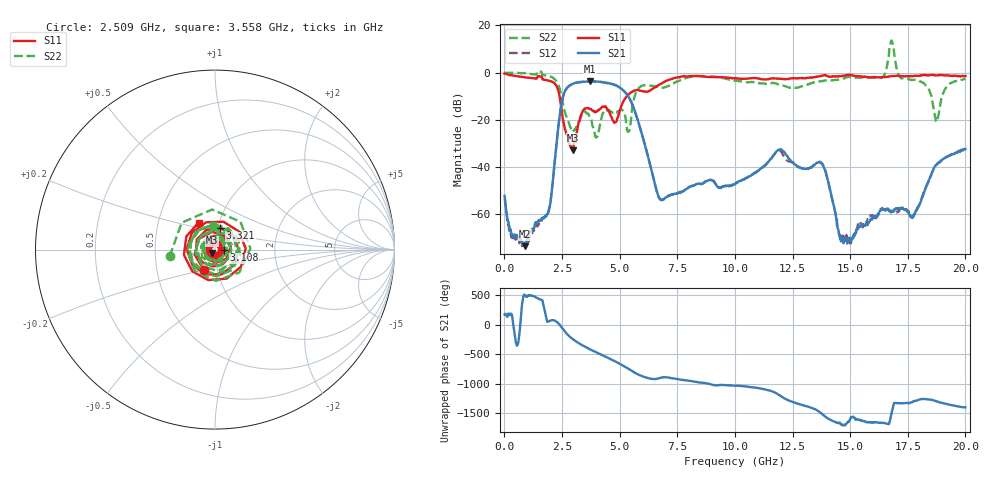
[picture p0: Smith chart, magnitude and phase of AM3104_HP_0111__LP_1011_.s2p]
!Created with skrf (http://scikit-rf.org).
# Hz S RI R 50.0
!freq ReS11 ImS11 ReS21 ImS21 ReS12 ImS12 ReS22 ImS22
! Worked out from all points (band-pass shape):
!   1601 points, 10 MHz to 20 GHz, reference 50 ohm
!   highest |S21| = -3.67 dB at 3.708 GHz (marker M1); lowest = -73.5 dB at 897.1 MHz (marker M2)
!   |S21| within 3 dB of the highest: 2.7 GHz to 5.061 GHz (2.362 GHz wide, 60.9 % of centre)
!   lowest |S11| = -32.8 dB at 2.971 GHz (marker M3), VSWR 1.05, Z = 48.5 - j1.68 ohm
!   |S11| at or under -10 dB: 2.394 GHz to 5.307 GHz (2.912 GHz wide, 75.6 % of centre)
!   |S22| runs from -27.5 to 13.6 dB; largest |S21 - S12| = 0.054
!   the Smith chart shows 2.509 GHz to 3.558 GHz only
!   S11 on the Smith chart (normalised r, x): 2.509 GHz: 0.86, -0.20; 3.108 GHz: 1.10, -0.01; 3.321 GHz: 1.03, +0.25; 3.558 GHz: 0.80, +0.25
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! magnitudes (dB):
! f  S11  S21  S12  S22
! 10 MHz  -0.3  -52.2  -53.4  0.0
! 897.1 MHz  -1.9  -73.5  -72.3  -0.2
! 1.922 GHz  -3.4  -58.4  -58.8  -1.4
! 2.509 GHz  -17.7  -11.6  -11.7  -11.8
! 2.971 GHz  -32.8  -4.7  -4.7  -25.0
! 3.108 GHz  -26.2  -4.2  -4.2  -23.1
! 3.321 GHz  -18.2  -3.9  -4.0  -18.7
! 3.346 GHz  -17.6  -3.9  -4.0  -18.0
! 3.558 GHz  -15.1  -3.8  -3.8  -17.2
! 3.708 GHz  -15.3  -3.7  -3.7  -18.9
! 5.395 GHz  -9.2  -10.3  -10.4  -24.9
! 5.795 GHz  -7.3  -20.4  -20.4  -7.0
! 6.682 GHz  -5.3  -52.3  -52.5  -6.2
! 10.01 GHz  -2.5  -47.2  -47.2  -3.4
! 11.93 GHz  -2.5  -32.5  -32.8  -5.1
! 13.34 GHz  -2.1  -39.9  -40.0  -4.4
! 13.87 GHz  -1.1  -40.2  -39.8  -3.4
! 14.67 GHz  -1.4  -70.0  -69.9  -2.6
! 16.68 GHz  -1.6  -58.0  -58.5  7.2
! 17.73 GHz  -1.4  -61.4  -60.4  -3.1
! 18.75 GHz  -1.2  -38.9  -38.9  -20.9
! 20 GHz  -1.4  -32.3  -31.7  -2.6
